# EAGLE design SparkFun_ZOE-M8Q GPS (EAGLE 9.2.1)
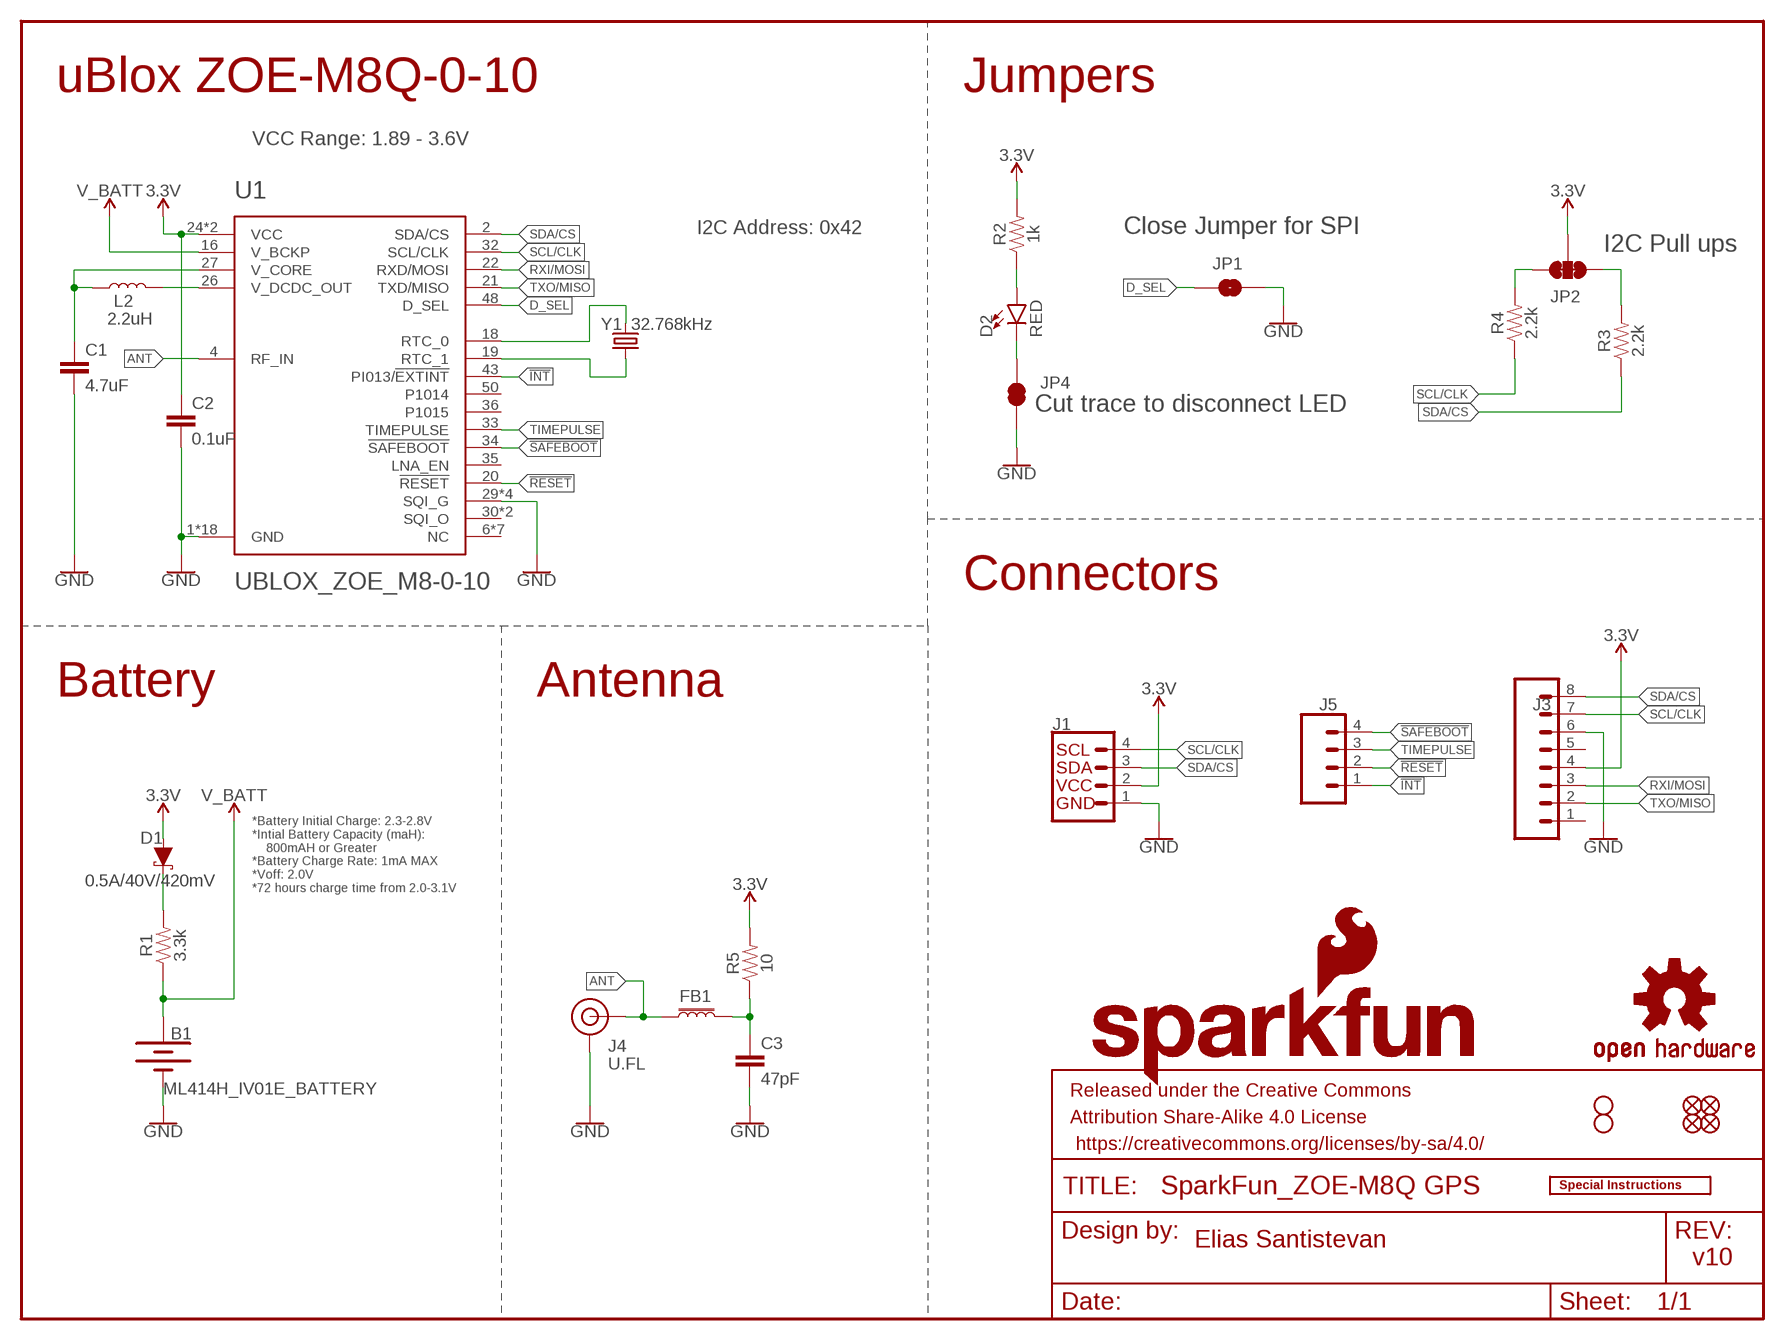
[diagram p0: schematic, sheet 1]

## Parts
B1  ML414H_IV01E_BATTERY  [ML414H_IV01E]
C1  4.7uF  4.7UF-0603-6.3V-(10%)  [0603]
C2  0.1uF  0.1UF-0603-25V-(+80/-20%)  [0603]
C3  47pF  47PF-0603-50V-5%  [0603]
D1  0.5A/40V/420mV  DIODE-SCHOTTKY-PMEG4005EJ  [SOD-323]
D2  RED  LED-RED0603  [LED-0603]
FB1  FERRITE_BEAD-120_OHM-0402  [0402]
FD1  FIDUCIALUFIDUCIAL  [FIDUCIAL-MICRO]
FD2  FIDUCIALUFIDUCIAL  [FIDUCIAL-MICRO]
FD3  FIDUCIALUFIDUCIAL  [FIDUCIAL-MICRO]
FD4  FIDUCIALUFIDUCIAL  [FIDUCIAL-MICRO]
FRAME1  FRAME-LETTER  [CREATIVE_COMMONS]
H2  STAND-OFFTIGHT  [STAND-OFF-TIGHT]
H3  STAND-OFFTIGHT  [STAND-OFF-TIGHT]
J1  QWIIC_CONNECTORJS-1MM  [JST04_1MM_RA]
J3  CONN_08NO_SILK_FEMALE_PTH  [1X08_NO_SILK]
J4  U.FL  U.FL2PIN  [U.FL]
J5  CONN_041X04_NO_SILK  [1X04_NO_SILK]
JP1  JUMPER-SMT_2_NO_SILK  [SMT-JUMPER_2_NO_SILK]
JP2  JUMPER-SMT_3_2-NC_TRACE_SILK  [SMT-JUMPER_3_2-NC_TRACE_SILK]
JP4  JUMPER-SMT_2_NC_TRACE_SILK  [SMT-JUMPER_2_NC_TRACE_SILK]
L2  2.2uH  2.2μH_SHIELDED_INDUCTOR  [0806]
LOGO1  SFE_LOGO_NAME_FLAME.1_INCH  [SFE_LOGO_NAME_FLAME_.1]
LOGO2  OSHW-LOGOS  [OSHW-LOGO-S]
LOGO3  SFE_LOGO_FLAME.1_INCH  [SFE_LOGO_FLAME_.1]
LOGO4  SPECIAL_INSTRUCTIONS-ORDERING  [ORDERING_INSTRUCTIONS]
R1  3.3k  3.3KOHM-0603-1/10W-1%  [0603]
R2  1k  1KOHM-0603-1/10W-1%  [0603]
R3  2.2k  2.2KOHM-0603-1/10W-1%  [0603]
R4  2.2k  2.2KOHM-0603-1/10W-1%  [0603]
R5  10  10OHM-0603-1/10W-1%  [0603]
U1  UBLOX_ZOE_M8-0-10  [UBLOX_ZOE_M8-0-10]
Y1  32.768kHz  CRYSTAL-32.768KHZSMD-3.2X1.5  [CRYSTAL-SMD-3.2X1.5MM]

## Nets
3.3V: C2.1 D1.A J1.2 J3.4 JP2.2 R2.2 R5.2 U1.24(VCC) U1.25(VCC)
!INT: J5.1 U1.43(PI013/!EXTINT)
!RESET: J5.2 U1.20(!RESET)
!SAFEBOOT: J5.4 U1.34(!SAFEBOOT)
ANT: FB1.1 J4.FEED(SIGNAL) U1.4(RF_IN)
D_SEL: JP1.1 U1.48(D_SEL)
GND: B1.- C1.2 C2.2 C3.2 J1.1 J3.6 J4.1(GND) J4.2(GND) JP1.2 JP4.1 U1.1(GND) U1.3(GND) U1.5(GND) U1.7(GND) U1.8(GND) U1.9(GND) U1.10(GND) U1.11(GND) U1.12(GND) U1.17(GND) U1.23(GND) U1.29(SQI_G) U1.31(SQI_G) U1.37(GND) U1.38(GND) U1.39(GND) U1.40(GND) U1.41(GND) U1.44(GND) U1.46(SQI_G) U1.47(SQI_G) U1.49(GND)
N$1: JP2.1 R3.2
N$2: D1.C R1.2
N$3: JP2.3 R4.2
N$4: D2.A R2.1
N$6: C1.1 L2.1 U1.27(V_CORE)
N$7: L2.2 U1.26(V_DCDC_OUT)
N$8: D2.C JP4.2
N$9: C3.1 FB1.2 R5.1
N$13: U1.18(RTC_0) Y1.P$2
N$15: U1.19(RTC_1) Y1.P$1
RXI/MOSI: J3.3 U1.22(RXD/MOSI)
SCL/CLK: J1.4 J3.7 R4.1 U1.32(SCL/CLK)
SDA/CS: J1.3 J3.8 R3.1 U1.2(SDA/CS)
TIMEPULSE: J5.3 U1.33(TIMEPULSE)
TXO/MISO: J3.2 U1.21(TXD/MISO)
V_BATT: B1.+ R1.1 U1.16(V_BCKP)
Unconnected: J3.1 J3.5 U1.6(NC) U1.13(NC) U1.14(NC) U1.15(NC) U1.28(NC) U1.30(SQI_O) U1.35(LNA_EN) U1.36(P1015) U1.42(NC) U1.45(SQI_O) U1.50(P1014) U1.51(NC)

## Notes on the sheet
- uBlox ZOE-M8Q-0-10 | Jumpers
- VCC Range: 1.89 - 3.6V
- I2C Address: 0x42 | Close Jumper for SPI
- I2C Pull ups
- Cut trace to disconnect LED
- Connectors
- Battery | Antenna
- *Battery Initial Charge: 2.3-2.8V
  *Intial Battery Capacity (maH): 
      800mAH or Greater
  *Battery Charge Rate: 1mA MAX
  *Voff: 2.0V
  *72 hours charge time from 2.0-3.1V
- Elias Santistevan
- v10

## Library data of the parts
B1 = SparkFun-Batteries:ML414H_IV01E_BATTERY: SEIKO ML414H-IV01E Reflowable Lithium Battery; PROD_ID: BATT-14267
C1 = SparkFun-Capacitors:4.7UF: 4.7µF ceramic capacitors; PROD_ID: CAP-08280
C2 = SparkFun-Capacitors:0.1UF: 0.1µF ceramic capacitors; PROD_ID: CAP-00810
C3 = SparkFun-Capacitors:47PF: 47pF ceramic capacitors; PROD_ID: CAP-08913
D1 = SparkFun-DiscreteSemi:DIODE-SCHOTTKY: Schottky diode; PROD_ID: DIO-10955
D2 = SparkFun-LED:LED-RED: Red SMD LED; PROD_ID: DIO-00819
FB1 = SparkFun-Coils:FERRITE_BEAD-120_OHM: Ferrite Bead (blocks, cores, rings, chokes, etc.); MFG_PART: BLM15HB121SN1D; PROD_ID: NDUC-14206
FD1-FD4 = SparkFun-Aesthetics:FIDUCIAL: Fiducial Alignment Points
FRAME1 = SparkFun-Aesthetics:FRAME-LETTER: Schematic Frame - Letter
H2 H3 = SparkFun-Hardware:STAND-OFF: Stand Off
J1 = SparkFun-Connectors:QWIIC_CONNECTOR: SparkFun I2C Standard Qwiic Connector An SMD 1mm pitch JST connector makes it easy and quick (get it? Qwiic?) to connect I2C devices to each other. The Qwiic system enables fast and solderless connection between popular platforms and various sensors and actuators. We carry 200mm, 100mm, 50mm, and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; PROD_ID: CONN-13694
J3 = SparkFun-Connectors:CONN_08: Multi connection point. Often used as Generic Header-pin footprint for 0.1 inch spaced/style header connections On any of the 0.1 inch spaced packages, you can populate with these: Break Away Headers - Straight (PRT-00116) Break Away Male Headers - Right Angle (PRT-00553) Female Headers (PRT-00115)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; PROD_ID: CONN-08438
J4 = SparkFun-Connectors:U.FL2PIN: SMD Antenna Connector - U.FL; PROD_ID: CONN-09193; SF_ID: WRL-09144
J5 = SparkFun-Connectors:CONN_04: Multi connection point. Often used as Generic Header-pin footprint for 0.1 inch spaced/style header connections On any of the 0.1 inch spaced packages, you can populate with these: Break Away Headers - Straight (PRT-00116) Break Away Male Headers - Right Angle (PRT-00553) Female Headers (PRT-00115)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; PROD_ID: CONN-09696
JP1 = SparkFun-Jumpers:JUMPER-SMT_2_NO: Normally open jumper
JP2 = SparkFun-Jumpers:JUMPER-SMT_3_2-NC_TRACE: Normally closed trace jumper (2 of 2 connections) This jumper has a trace between all three pads so they are normally closed (NC). Use a razor knife to open the connection(s). For best results follow the IPC guidelines for cutting traces: Cutout at least 0.063 mm (0.005 in). Remove all loose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
JP4 = SparkFun-Jumpers:JUMPER-SMT_2_NC_TRACE: Normally closed trace jumper
L2 = SparkFun-Coils:2.2μH_SHIELDED_INDUCTOR: Murata 2.2uH Inductor; PROD_ID: NDUC-14257
LOGO1 = SparkFun-Aesthetics:SFE_LOGO_NAME_FLAME: SparkFun Font Logo w/ Flame
LOGO2 = SparkFun-Aesthetics:OSHW-LOGO: Open-Source Hardware (OSHW) Logo
LOGO3 = SparkFun-Aesthetics:SFE_LOGO_FLAME: SparkFun Flame Logo
LOGO4 = SparkFun-Aesthetics:SPECIAL_INSTRUCTIONS: Special Ordering/Production Instructions Alert
R1 = SparkFun-Resistors:3.3KOHM: 3.3kΩ resistor; PROD_ID: RES-07851
R2 = SparkFun-Resistors:1KOHM: 1kΩ resistor; PROD_ID: RES-07856
R3 R4 = SparkFun-Resistors:2.2KOHM: 2.2kΩ resistor; PROD_ID: RES-08272
R5 = SparkFun-Resistors:10OHM: 10Ω resistor; PROD_ID: RES-12581
U1 = SparkFun-GPS:UBLOX_ZOE_M8-0-10: UBLOX ZOE-M8Q-0-10 u-blox ZOE-M8 standard precision GNSS SiP (System in Package) modules feature the high performance u-blox M8 GNSS engine. ZOE-M8’s ultra-miniature form factor integrates a complete GNSS receiver including SAW filter, LNA and TCXO. Handles all GNSS systems and can simulatenously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; PROD_ID: IC-14251
Y1 = SparkFun-Clocks:CRYSTAL-32.768KHZ: 32.768kHz Crystal; PROD_ID: XTAL-13062

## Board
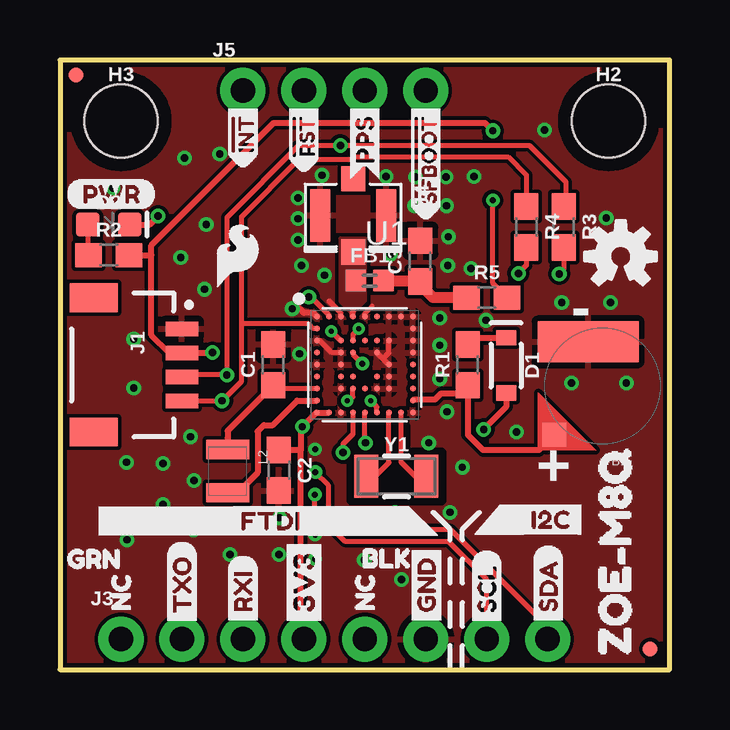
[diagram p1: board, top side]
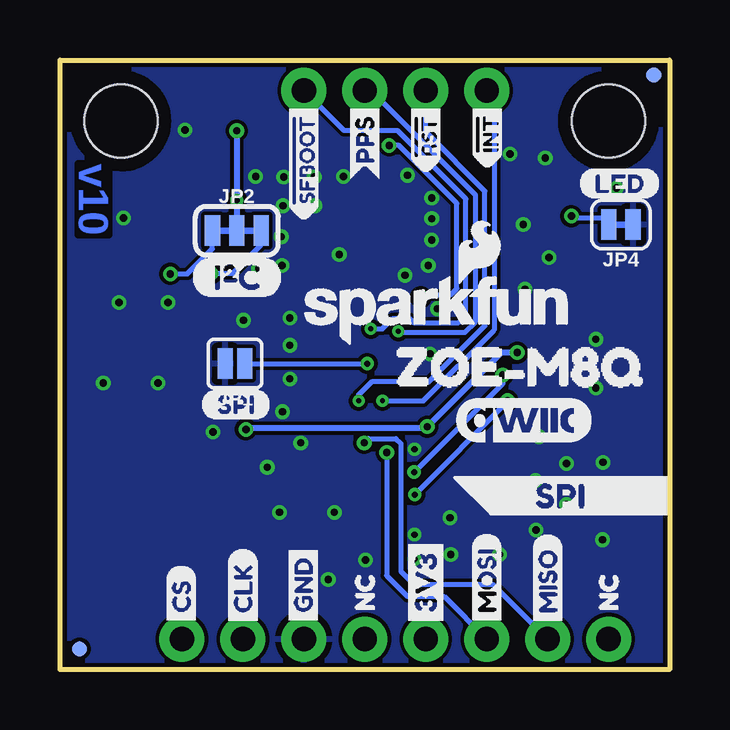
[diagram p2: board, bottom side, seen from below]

Size 25.4 x 25.4 mm. Coordinates in mm from the lower left corner, seen from the top.
Outline: 0,0 25.4,0 25.4,25.4 0,25.4 0,0
Copper layers (1*16): Top 0.035mm / dielectric 1.5mm / Bottom 0.035mm
Design rules "SparkFun-2-layer-TIGHT *": minimum track width 7mil, minimum drill 15mil, track to track 6mil, track to pad 6mil, pad to pad 6mil, via to via 6mil, smd to smd 6mil, copper to edge 7mil, drill to drill 7mil, minimum pad ring 7mil, minimum via ring 6mil, stop-mask expansion 4mil, vias tented up to drill 25mil, thermal gap 10mil
tRestrict: 7 lines

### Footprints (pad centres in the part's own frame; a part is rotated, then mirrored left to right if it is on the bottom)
ML414H_IV01E = smd 1 x 1: + 2.022,2.032 | smd 4.2 x 1.7: - 0.6,-1.85
0603 = smd 1.1 x 1: 1 -0.85,0; 2 0.85,0
SOD-323 = smd 0.63 x 0.83: A 1.15,0; C -1.15,0
LED-0603 = smd 1 x 1: A -0.877,0; C 0.877,0
0402 = smd 0.85 x 0.9: 1 -0.58,0; 2 0.58,0
FIDUCIAL-MICRO = smd 0.635 x 0.635: 1 0,0
STAND-OFF-TIGHT = hole 3.048: 0,0
JST04_1MM_RA = smd 0.6 x 1.35: 1 -1.5,0; 2 -0.5,0; 3 0.5,0; 4 1.5,0 | smd 1.2 x 2: NC1 2.8,-3.675; NC2 -2.8,-3.675
1X08_NO_SILK = drill 1.016 pad 1.88: 1 0,0; 2 2.54,0; 3 5.08,0; 4 7.62,0; 5 10.16,0; 6 12.7,0; 7 15.24,0; 8 17.78,0
U.FL = smd 2.2 x 0.85: 1 0,1.375; 2 0,-1.375 | smd 1.05 x 1: FEED 1.525,0; NC -1.525,0
1X04_NO_SILK = drill 1.016 pad 1.88: 1 0,0; 2 2.54,0; 3 5.08,0; 4 7.62,0
SMT-JUMPER_2_NO_SILK = smd 0.635 x 1.27: 1 -0.406,0; 2 0.406,0
SMT-JUMPER_3_2-NC_TRACE_SILK = smd 0.635 x 1.27: 1 -1.016,0; 2 0,0; 3 1.016,0
SMT-JUMPER_2_NC_TRACE_SILK = smd 0.635 x 1.27: 1 -0.508,0; 2 0.508,0
0806 = smd 0.8 x 1.8: 1 -1.3,0; 2 0.5,0
UBLOX_ZOE_M8-0-10 = smd 0.25 x 0.25: 1 -1.996,2.004; 2 -1.496,2.004; 3 -0.996,2.004; 4 -0.496,2.004; 5 0.004,2.004; 6 0.504,2.004; 7 1.004,2.004; 8 1.504,2.004; 9 2.004,2.004; 10 2.004,1.504; 11 2.004,1.004; 12 2.004,0.504; 13 2.004,0.004; 14 2.004,-0.496; 15 2.004,-0.996; 16 2.004,-1.496; 17 2.004,-1.996; 18 1.504,-1.996; 19 1.004,-1.996; 20 0.504,-1.996; 21 0.004,-1.996; 22 -0.496,-1.996; 23 -0.996,-1.996; 24 -1.496,-1.996; 25 -1.996,-1.996; 26 -1.996,-1.496; 27 -1.996,-0.996; 28 -1.996,-0.496; 29 -1.996,0.004; 30 -1.996,0.504; 31 -1.996,1.004; 32 -1.996,1.504; 33 -0.996,1.004; 34 -0.496,1.004; 35 0.004,1.004; 36 0.504,1.004; 37 1.004,1.004; 38 1.004,0.004; 39 1.004,-0.496; 40 1.004,-0.996; 41 0.504,-0.996; 42 0.004,-0.996; 43 -0.496,-0.996; 44 -0.996,-0.996; 45 -0.996,-0.496; 46 -0.996,0.004; 47 -0.996,0.504; 48 -0.496,0.504; 49 0.504,0.504; 50 0.504,-0.496; 51 -0.496,-0.496
CRYSTAL-SMD-3.2X1.5MM = smd 1 x 1.8: P$1 -1.25,0; P$2 1.25,0

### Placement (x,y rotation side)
B1  22.61,11.81 180 top
C1  8.89,12.7 90 top
C2  9.12,8.31 270 top
C3  15.01,17.02 90 top
D1  18.59,12.67 270 top
D2  2.03,18.54 0 top
FB1  12.9,16.21 0 top
FD1  0.66,24.77 0 top
FD2  24.59,0.86 0 bottom
FD3  0.66,24.77 0 bottom
FD4  24.59,0.86 0 top
FRAME1  not placed on the board
H2  22.86,22.86 0 top
H3  2.54,22.86 0 top
J1  5.08,12.7 270 top
J3  2.54,1.27 0 top
J4  12.22,18.92 270 top
J5  7.62,24.13 0 top
JP1  18.11,12.75 180 bottom
JP2  18.03,18.29 0 bottom
JP4  2.03,18.54 180 bottom
L2  6.99,7.87 270 top
LOGO1  9.65,14.99 0 bottom
LOGO2  23.36,17.21 0 top
LOGO3  7.39,17.26 0 top
LOGO4  not placed on the board
R1  16.99,12.7 90 top
R2  2.03,17.27 0 top
R3  20.98,18.44 270 top
R4  19.43,18.44 270 top
R5  17.78,15.49 0 top
U1  12.7,12.7 0 top
U$1  [3V3-03]  10.16,1.57 90 top
U$2  [SDA0]  20.35,1.7 90 top
U$3  [SCL0]  17.78,1.68 90 top
U$4  [GND0]  15.27,1.7 90 top
U$5  [CS0]  20.35,1.68 90 bottom
U$6  [MISO0]  5.08,1.65 90 bottom
U$7  [GND0]  15.27,1.7 90 bottom
U$8  [CLK0]  17.78,1.68 90 bottom
U$9  [SPI0]  6.49,7.24 0 bottom
U$10  [3V3-03]  10.16,1.57 90 bottom
U$11  [#INT0]  7.62,20.73 90 top
U$12  [#RST0]  10.16,20.57 90 top
U$13  [PPS0]  12.7,20.4 90 bottom
U$14  [#SFBOOT0]  15.24,18.59 90 top
U$15  [TXO0]  5.08,1.65 90 top
U$16  [ZOE#M8Q0]  12.75,12.62 0 bottom
U$17  [SPI0]  19.52,11.04 0 bottom
U$18  [#INT0]  7.59,20.73 90 bottom
U$19  [RXI0]  7.62,1.7 90 top
U$20  [BLK0]  11.9,4.64 0 top
U$21  [#RST0]  10.16,20.57 90 bottom
U$22  [NC0]  12.7,1.78 90 top
U$23  [PPS0]  12.7,20.4 90 top
U$24  [#SFBOOT0]  15.24,18.59 90 bottom
U$25  [LED0]  3.81,20.26 0 bottom
U$26  [PWR-()-03]  0.25,19.81 0 top
U$27  [MOSI0]  7.62,1.68 90 bottom
U$28  [FTDI0]  6.83,6.2 0 top
U$29  [I2C0]  18.92,6.25 0 top
U$30  [ZOE#M8Q0]  23.11,-0.51 90 top
U$31  [GRN0]  -0.38,4.62 0 top
U$32  [I_SUPER2_C-()-04]  19.92,16.35 0 bottom
U$33  [NC0]  2.54,1.78 90 top
U$34  [NC0]  12.7,1.78 90 bottom
U$35  [NC0]  2.54,1.78 90 bottom
U$36  [QWIIC_COPYRIGHT_SMALL]  6.1,10.41 0 bottom
Y1  14.02,8.05 0 top

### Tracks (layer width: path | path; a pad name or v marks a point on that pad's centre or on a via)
3.3V  (via drill 0.25, 0.3)
  Top 0.203: R5.2 18.03,16.09 v18.03,19.56
  Top 0.254: U1.24 U1.25 10.68,10.7 v10.1,10.12 10.03,10.06 10.03,9.14 | v6.35,13.21 J1.2 4.55,13.2 3.81,13.94 3.81,17.27 | D1.A 18.59,10.95 v17.65,10.01 | v18.03,22.45 17.7,22.78 8.91,22.78 3.81,17.68 3.81,17.27 | R2.2 3.81,17.27 | 10.03,9.14 10.03,1.4 J3.4 | 10.03,9.14 9.13,9.14 C2.1
  Bottom 0.254: v6.35,13.21 7.01,13.21 v10.1,10.12 10.16,10.06 17.6,10.06 v17.65,10.01 | v18.03,22.45 v18.03,19.56 JP2.2
!INT  (via drill 0.2)
  Top 0.203: v11.96,11.2 12.04,11.2 12.2,11.37 U1.43
  Bottom 0.203: v11.96,11.2 10.26,11.2 7.32,14.15 7.32,23.82 J5.1
!RESET  (via drill 0.2)
  Top 0.203: U1.20 13.2,10.95 v12.95,11.2
  Bottom 0.203: v12.95,11.2 12.95,11.46 12.42,11.99 10.03,11.99 7.7,14.33 7.7,19.94 10.16,22.4 J5.2
!SAFEBOOT  (via drill 0.2)
  Top 0.203: v12.45,14.2 12.2,13.96 U1.34
  Bottom 0.203: J5.4 13.56,22.45 11.33,22.45 8.48,19.61 8.48,14.76 8.79,14.45 10.67,14.45 10.85,14.63 11.53,14.63 11.96,14.2 v12.45,14.2
ANT
  Top 0.254: U1.4 12.2,14.95
  pour Top (isolate 0.152, no thermals): 11.68,17.14 11.68,15.29 12.09,14.88 12.24,14.88 12.73,15.37 12.73,17.98 11.71,17.98 11.68,17.98
D_SEL  (via drill 0.25)
  Top 0.203: U1.48 12.2,13.14 v12.6,12.75
  Bottom 0.203: JP1.1 v12.6,12.75
GND  (via drill 0.25 pad 0.25, 0.3)
  Top 0.203: U1.47 11.33,13.2 10.83,13.7 U1.31 | U1.49 13.46,12.95 | 13.46,12.95 U1.38 | 13.46,12.95 13.7,13.2 U1.37 | U1.3 11.7,14.86 11.21,15.36 | U1.5 12.7,14.85 13,15.14
  Top 0.254: U1.1 10.55,14.86 10.16,14.86 9.98,15.04 v9.68,15.04
  other vias: 22.94,15.29 20.19,22.48 4.29,6.88 6.1,18.54 5.18,21.31 22.76,18.82 2.77,8.64 15.37,9.45 5.44,9.7 11.02,16.43 9.91,17.9 9.91,19.65 10.92,20.6 13.59,20.55 14.78,19.33 16.1,19.33 16.08,20.52 14.81,20.52 10.06,16.84 9.91,18.79 17.25,20.55 16.18,18.03 16.15,16.84 17.12,16.71 5.59,7.87 4.29,8.59 5.03,17.17 6.02,15.85 6.65,21.49 2.21,20.07 16.76,8.43 3.07,11.73 2.79,5.41 15.82,13.51 15.82,12.12 15.82,14.66 9.98,13.16 9.14,6.32 9.12,4.8 5.56,5.82 21.31,11.94 23.6,11.94 12.67,4.57 3.07,13.77 7.09,4.8 16.13,10.74 20.9,15.29 19.02,9.91 17.75,14.55 13.97,6.55 14.22,3.76 10.63,9.18 10.63,5.63 10.63,4.61 16.26,6.55 13.77,17.3
  pour Top (isolate 0.152, rank 4): 0,25.4 0,0 25.4,0 25.4,25.4
  pour Bottom (isolate 0.152, rank 4): 0,25.4 0,0 25.4,0 25.4,25.4
N$1  (via drill 0.3)
  Top 0.203: R3.2 20.98,16.66 v20.8,16.48
  Bottom 0.203: v20.8,16.48 20.09,16.48 19.05,17.53 JP2.1
N$2
  Top 0.254: D1.C 18.57,13.8 17.25,13.8 R1.2
N$3  (via drill 0.3)
  Top 0.203: R4.2 19.43,16.84 v19.1,16.51
  Bottom 0.203: v19.1,16.51 18.21,16.51 17.02,17.7 JP2.3
N$4
  Top 0.203: D2.A 1.16,17.3 R2.1
N$6
  Top 0.203: C1.1 9.08,11.66 9.12,11.7 U1.27
  Top 0.254: C1.1 6.99,9.95 6.99,9.65 L2.1
N$7
  Top 0.254: U1.26 9.88,11.2 8.87,10.19 8.49,10.19 8.23,9.93 8.23,8.2 7.4,7.37 L2.2
N$8  (via drill 0.3)
  Top 0.254: D2.C 3.73,18.54 v4.09,18.9
  Bottom 0.203: v4.09,18.9 3.99,18.8 2.79,18.8 JP4.2
N$9
  Top 0.457: FB1.2 14.83,16.2 15.01,16.03 | 15.01,16.03 C3.1 | R5.1 15.54,15.49 15.01,16.03
N$13
  Top 0.203: Y1.P$2 14.81,8.05 14.2,8.66 U1.18
N$15
  Top 0.203: Y1.P$1 13.13,8.05 13.7,8.62 U1.19
RXI/MOSI  (via drill 0.3)
  Top 0.203: U1.22 12.2,9.82 11.79,9.4 v11.79,9.04
  Bottom 0.203: v11.79,9.04 11.79,3.91 10.92,3.05 9.4,3.05 J3.3
SCL/CLK  (via drill 0.25, 0.3)
  Top 0.203: 7.57,14.35 7.57,12.01 v6.75,11.2 J1.4 | 7.57,14.35 7.57,18.87 9.96,21.26 12.14,21.26 12.24,21.36 18.67,21.36 19.43,20.6 R4.1 | U1.32 10.56,14.2 10.36,14.4 7.62,14.4 7.57,14.35 | J3.7 17.78,3.76 16.2,5.33 11.89,5.33 10.62,6.61 v10.62,7.29
  Bottom 0.203: v10.62,7.29 6.75,11.15 v6.75,11.2
SDA/CS  (via drill 0.25, 0.3)
  Top 0.203: J1.3 5.16,12.28 v6.95,12.28 v6.96,12.28 6.96,18.85 9.96,21.84 v11.68,21.84 19.56,21.84 21.08,20.32 21.08,19.39 R3.1 | U1.2 11.2,14.78 10.46,15.52 v10.36,15.52 | J3.8 20.32,1.78 16.26,5.84 11.94,5.84 11.18,6.6 11.18,7.7 v10.64,8.23
  Bottom 0.203: v10.36,15.52 10.26,15.62 9.12,15.62 8.87,15.88 8.87,19.43 11.28,21.84 v11.68,21.84 | v10.64,8.23 6.95,11.92 v6.95,12.28
TIMEPULSE  (via drill 0.2)
  Top 0.203: U1.33 v11.31,14.1 v11.3,14.1
  Bottom 0.203: v11.3,14.1 11.25,14.05 8.53,14.05 8.08,14.5 8.08,19.76 12.45,24.13 J5.3
TXO/MISO  (via drill 0.3)
  Top 0.203: v12.72,9.45 12.7,9.47 U1.21
  Bottom 0.203: v12.72,9.45 12.55,9.63 11.4,9.63 11.2,9.42 11.2,4.09 10.67,3.56 7.37,3.56 J3.2
V_BATT
  Top 0.254: U1.16 14.76,11.26 15.63,11.26 15.89,11.51 16.99,11.51 | R1.1 16.99,11.51 | 16.99,11.51 16.99,9.78 17.63,9.14 19.95,9.14 B1.+

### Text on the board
Bottom: v10
tPlace: - | +
Measures: Units in Inches
tDocu: Elias Santistevan | 0.8mm Board Thickness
